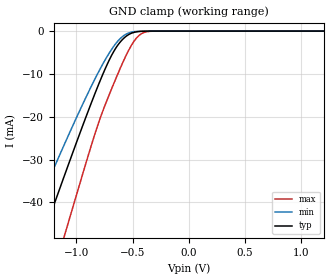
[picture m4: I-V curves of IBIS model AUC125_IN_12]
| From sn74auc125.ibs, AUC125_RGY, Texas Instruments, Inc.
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[Model]   AUC125_IN_12
Model_type  Input
Vinl=0.385
Vinh=0.845
| variable   typ   min   max
C_comp   2.40pF   2.03pF   2.74pF
[Temperature Range]   40   100   -40
| Ambient temperature   25   85   -40
[Voltage range]   1.2   1.1   1.3
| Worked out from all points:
|   GND clamp passes 1 mA (typ) near -0.55 V on its own axis
[GND Clamp]
| AUC125_IN_12
|   Voltage   I(typ)   I(min)   I(max)
-3.6V     -222.3mA   -186mA     -267.4mA
-1.45V    -59.26mA   -47.28mA   -78.52mA
-1.275V   -46.2mA    -36.55mA   -62.91mA
-1.11V    -34.05mA   -26.68mA   -48.18mA
-1.075V   -31.51mA   -24.62mA   -45.06mA
-835mV    -14.64mA   -11.21mA   -24.05mA
-695mV    -6.113mA   -4.618mA   -14.06mA
-575mV    -1.603mA   -998uA     -6.664mA
-500mV    -407.1uA   -201.5uA   -2.896mA
-440mV    -95.43uA   -45.01uA   -977.4uA
-320mV    -2.85uA    -1.742uA   -25.53uA
1.2V      133.3pA    223pA      123.7pA
